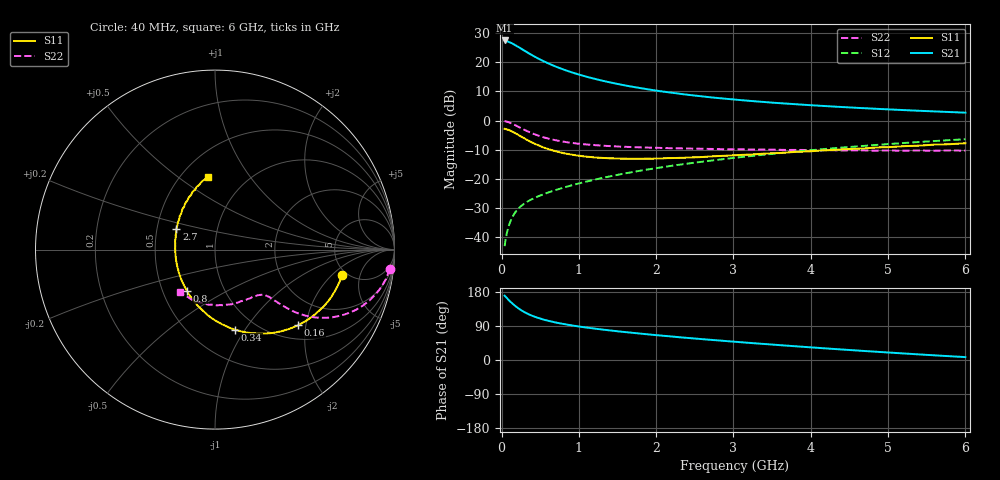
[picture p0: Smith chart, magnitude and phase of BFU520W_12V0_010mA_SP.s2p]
! Filename:  P:\Prog\Test\Noise\ATS_data\Testdata_Net\Run2\BFU520W_APM2013_06_A05_12p0V_010mA_SP_CM01_D.s2p
! Date/Time: Tue 26/Mar/2013 18:01:44
! BFU520W_APM2013_06_A05_12p0V_1to20mA_SP_CM01_Bias6_R.s2p
! MDIF S-parameter v. bias file
! BFU520W_APM2013_06_A05_12p0V_1to20mA_SP_CM01
! Date/time Thu Mar 21 16:35:01 2013
! VAR V_out= 12.0000
! VAR I_out= 9.9950
! VAR V_in= 0.8084
! VAR I_in= 0.1014
! Device data file deembeded for feedlines and parallel
! Original file: \Run2\BFU520W_APM2013_06_A05_12p0V_010mA_SP_CM01_R.s2p
! Feed-files: PR019V01_070313_Feed1.s2p, PR019V01_070313_Feed2.s2p
! Parallel-file: PR019V01_070313_Par.s2p
# MHz S MA R 50
!  Freq-MHz  S11-mag  S11-arg  S21-mag  S21-arg  S12-mag  S12-arg  S22-mag  S22-arg
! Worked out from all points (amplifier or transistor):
!   98 points, 40 MHz to 6 GHz, reference 50 ohm
!   highest |S21| = 27.4 dB at 40 MHz (marker M1)
!   |S21| within 3 dB of that: start of sweep to 265.5 MHz
!   unconditionally stable (mu >= 1): 1.515 GHz to 2.74 GHz
!   at 300 MHz: K = 0.50, MSG = 26.1 dB, |S12| = -28.4 dB
!   at 1.6 GHz: K = 1.00, MAG = 14.7 dB, |S12| = -18.1 dB
!   at 6 GHz: K = 0.88, MSG = 4.6 dB, |S12| = -6.4 dB
!   S11 on the Smith chart (normalised r, x): 40 MHz: 4.55, -2.67; 160 MHz: 1.30, -1.81; 340 MHz: 0.80, -0.90; 800 MHz: 0.66, -0.33; 2.7 GHz: 0.63, +0.15; 6 GHz: 0.67, +0.65
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40  0.7215 -11.2  23.56 169.9  0.007057 82.9  0.9787 -6.3
50  0.7174 -14.1  23.54 167.5  0.008667 82.0  0.9731 -8.0
100  0.6832 -27.6  22.04 156.9  0.01662 76.6  0.9279 -15.6
120  0.6645 -32.9  21.55 152.8  0.01948 74.5  0.906 -18.3
160  0.6261 -42.4  20.16 145.6  0.02473 71.0  0.8564 -22.9
200  0.5854 -51.0  18.78 139.1  0.0292 68.3  0.8044 -26.8
240  0.5448 -59.1  17.5 133.3  0.03314 66.3  0.7561 -29.9
280  0.5085 -66.3  16.22 128.3  0.03664 64.8  0.7107 -32.3
340  0.4598 -76.0  14.54 121.8  0.04123 63.4  0.6518 -35.0
380  0.4307 -81.8  13.52 118.2  0.04409 62.9  0.6177 -36.4
440  0.3951 -89.7  12.22 113.4  0.04815 62.5  0.5752 -37.7
550  0.3432 -102.1  10.31 106.3  0.05504 62.7  0.5138 -39.2
650  0.3113 -111.8  8.983 101.3  0.06137 63.2  0.4758 -39.8
800  0.2768 -124.6  7.504 95.1  0.07084 64.1  0.4359 -40.5
1050  0.2452 -142.2  5.881 87.0  0.08696 65.5  0.3951 -41.4
1500  0.2237 -166.7  4.24 75.8  0.1175 66.3  0.3601 -44.5
2050  0.2239 171.6  3.189 64.7  0.1566 65.5  0.3405 -50.3
2700  0.2428 152.3  2.508 53.3  0.2052 63.0  0.327 -60.0
3100  0.2579 142.3  2.237 46.9  0.2368 61.0  0.3217 -66.3
4100  0.305 123.2  1.801 31.9  0.319 54.3  0.31 -85.6
5200  0.364 106.2  1.513 17.3  0.4125 45.2  0.3042 -109.9
6000  0.4088 95.6  1.366 7.7  0.4788 37.7  0.3049 -129.9
